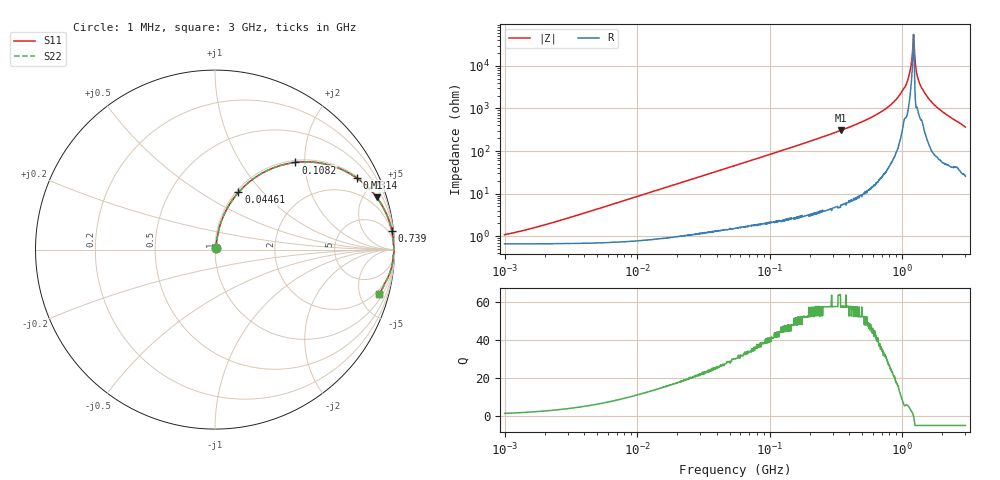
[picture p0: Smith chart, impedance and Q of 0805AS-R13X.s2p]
!s-Parameter Generated by FASTRON Sdn. Bhd.
!FASTRON P/N : 0805AS-R13X
!Keysight Technologies: E4991B_MY54100416_A.01.15
!Date: Mon Jun 15 12:52:20 2026
!Version  :Rev01  Mon Jun 15 12:52:20 2026
!Data & Calibration Information:
!Freq  S11  S21  S12  S22
!PortZ  Port1:50+j0  Port2:50+j0
!When reading reference impedance value at option line is always used.
! Remarks : This data is being provided solely for informational purposes.
# Hz S dB R 50
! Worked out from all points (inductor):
!   1601 points, 1 MHz to 3 GHz, reference 50 ohm
!   read as one part in series: L = 136 nH near 2.33 MHz
!   highest Q = 57.5 at 347.1 MHz (marker M1), where L = 142 nH
!   self-resonance near 1.213 GHz
!   S11 on the Smith chart (normalised r, x): 1 MHz: 1.01, +0.02; 44.61 MHz: 1.03, +0.74; 108.2 MHz: 1.04, +1.80; 231.4 MHz: 1.07, +3.93; 739 MHz: 2, +19; 3 GHz: 1.51, -7.29
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1000000  -39.40 52.1  -0.06 -0.5  -0.06 -0.5  -39.40 52.1
3804036  -29.60 76.4  -0.06 -1.9  -0.06 -1.9  -29.60 76.4
1.447069e7  -18.30 79.0  -0.14 -6.9  -0.14 -6.9  -18.30 79.0
4.461279e7  -9.25 67.7  -0.67 -20.2  -0.67 -20.2  -9.25 67.7
5.504702e7  -7.71 63.8  -0.94 -24.3  -0.94 -24.3  -7.71 63.8
1.081723e8  -3.60 47.3  -2.67 -41.3  -2.67 -41.3  -3.60 47.3
2.083556e8  -1.29 29.4  -6.19 -59.6  -6.19 -59.6  -1.29 29.4
2.314421e8  -1.06 26.8  -6.93 -62.2  -6.93 -62.2  -1.06 26.8
3.471137e8  -0.48 17.9  -10.30 -71.1  -10.30 -71.1  -0.48 17.9
7.38967e8  -0.08 6.0  -19.60 -82.2  -19.60 -82.2  -0.08 6.0
7.925923e8  -0.06 5.1  -21.00 -82.8  -21.00 -82.8  -0.06 5.1
9.302341e8  -0.04 3.1  -25.30 -83.3  -25.30 -83.3  -0.04 3.1
1.064802e9  -0.05 1.6  -30.80 -78.3  -30.80 -78.3  -0.05 1.6
1.125055e9  -0.03 1.0  -35.40 -77.0  -35.40 -77.0  -0.03 1.0
1.182785e9  -0.03 0.4  -43.00 -65.0  -43.00 -65.0  -0.03 0.4
1.212752e9  -0.02 0.1  -52.80 -26.6  -52.80 -26.6  -0.02 0.1
1.249715e9  -0.01 -0.4  -43.40 80.1  -43.40 80.1  -0.01 -0.4
1.294266e9  -0.03 -0.9  -35.80 79.3  -35.80 79.3  -0.03 -0.9
1.333714e9  -0.03 -1.3  -33.00 79.1  -33.00 79.1  -0.03 -1.3
1.526649e9  -0.05 -2.8  -26.10 81.3  -26.10 81.3  -0.05 -2.8
1.970482e9  -0.12 -6.4  -19.10 79.9  -19.10 79.9  -0.12 -6.4
3e9  -0.47 -15.0  -11.70 71.0  -11.70 71.0  -0.47 -15.0
